(* Logix 5000 AddOnInstructionDefinition export HI1769_AOI_INT; software revision 32.00; part 2 of 2 *)
(* tags used below, declared in another part *)
   Inp_hi1769 : HI:1769_xWS_ChannelNOCMD_r3:I:0;
   Out_hi1769 : HI:1769_xWS_Channel:O:0;
   cal_hi_cmd : BOOL;   // trigger the cal high command
   cal_low_cmd : BOOL;   // trigger the cal low command
   cmd_status : INT;
   cal_hi_ctrl : DINT;
   cal_lo_ctrl : DINT;
   CalHI_cmd_reset_timer : TIMER;
   CalLo_cmd_reset_timer : TIMER;
   Status_Return : HardyCmdResult;
(* HI1769_AOI_INT, continued *)

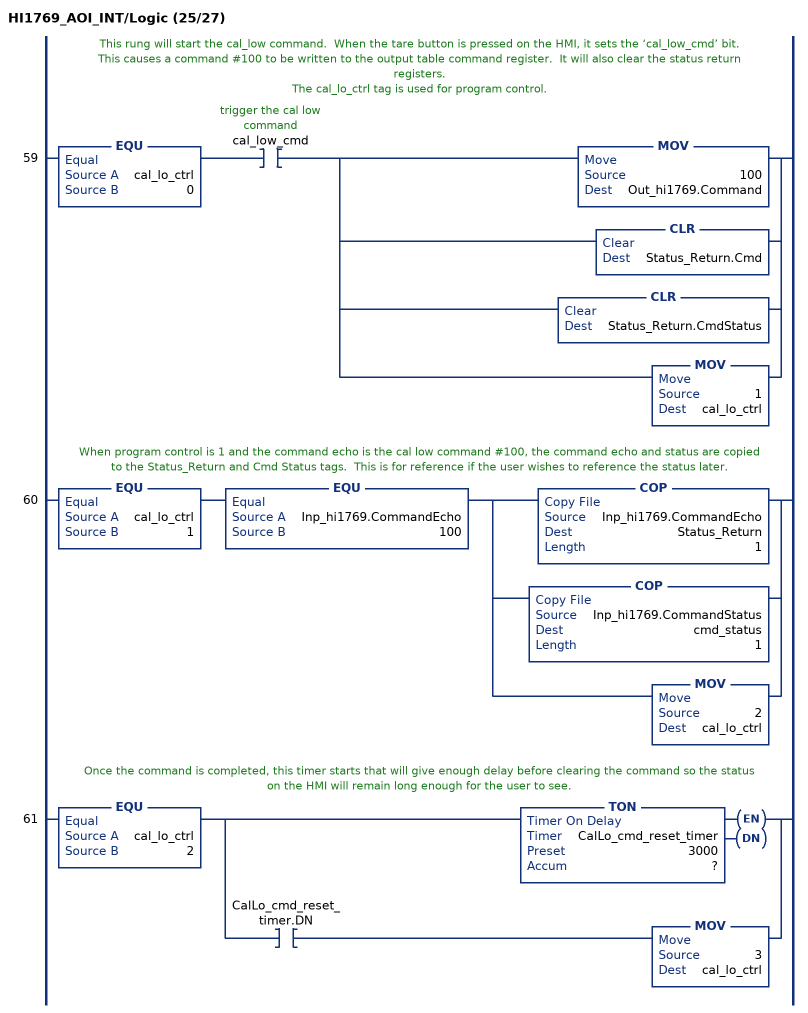
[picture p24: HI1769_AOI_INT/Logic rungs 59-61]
   // This rung will start the cal_low command.  When the tare button is pressed on the HMI, it sets the ‘cal_low_cmd’ bit.
   // This causes a command #100 to be written to the output table command register.  It will also clear the status return registers.
   // The cal_lo_ctrl tag is used for program control.
   59: EQU(cal_lo_ctrl,0)XIC(cal_low_cmd)[MOV(100,Out_hi1769.Command) ,CLR(Status_Return.Cmd) ,CLR(Status_Return.CmdStatus) ,MOV(1,cal_lo_ctrl) ];
   // When program control is 1 and the command echo is the cal low command #100, the command echo and status are copied to the Status_Return and Cmd Status tags.  This is for reference if the user wishes to reference the status later.
   60: EQU(cal_lo_ctrl,1)EQU(Inp_hi1769.CommandEcho,100)[COP(Inp_hi1769.CommandEcho,Status_Return,1) ,COP(Inp_hi1769.CommandStatus,cmd_status,1) ,MOV(2,cal_lo_ctrl) ];
   // Once the command is completed, this timer starts that will give enough delay before clearing the command so the status on the HMI will remain long enough for the user to see.
   61: EQU(cal_lo_ctrl,2)[TON(CalLo_cmd_reset_timer,?,?) ,XIC(CalLo_cmd_reset_timer.DN) MOV(3,cal_lo_ctrl) ];
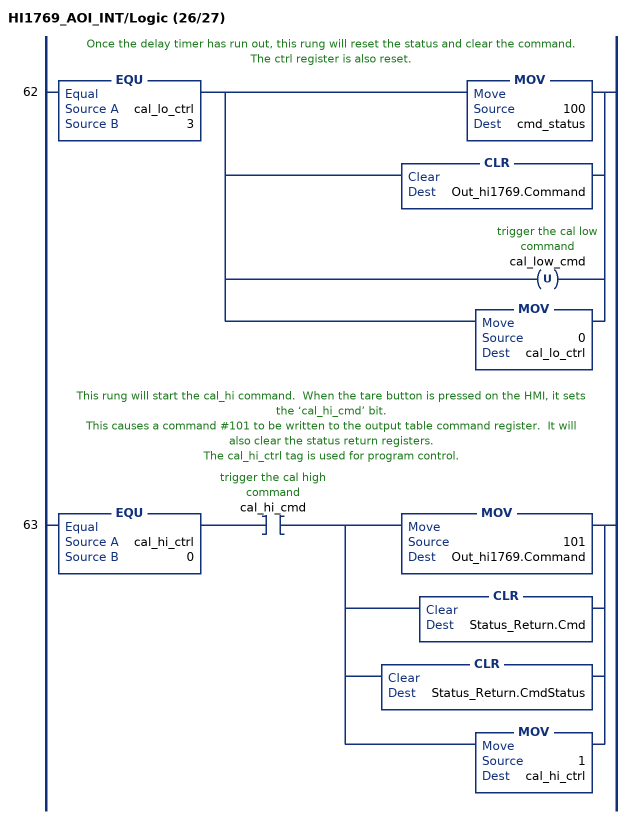
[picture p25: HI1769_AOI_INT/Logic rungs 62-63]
   // Once the delay timer has run out, this rung will reset the status and clear the command.
   // The ctrl register is also reset.
   62: EQU(cal_lo_ctrl,3)[MOV(100,cmd_status) ,CLR(Out_hi1769.Command) ,OTU(cal_low_cmd) ,MOV(0,cal_lo_ctrl) ];
   // This rung will start the cal_hi command.  When the tare button is pressed on the HMI, it sets the ‘cal_hi_cmd’ bit.
   // This causes a command #101 to be written to the output table command register.  It will also clear the status return registers.
   // The cal_hi_ctrl tag is used for program control.
   63: EQU(cal_hi_ctrl,0)XIC(cal_hi_cmd)[MOV(101,Out_hi1769.Command) ,CLR(Status_Return.Cmd) ,CLR(Status_Return.CmdStatus) ,MOV(1,cal_hi_ctrl) ];
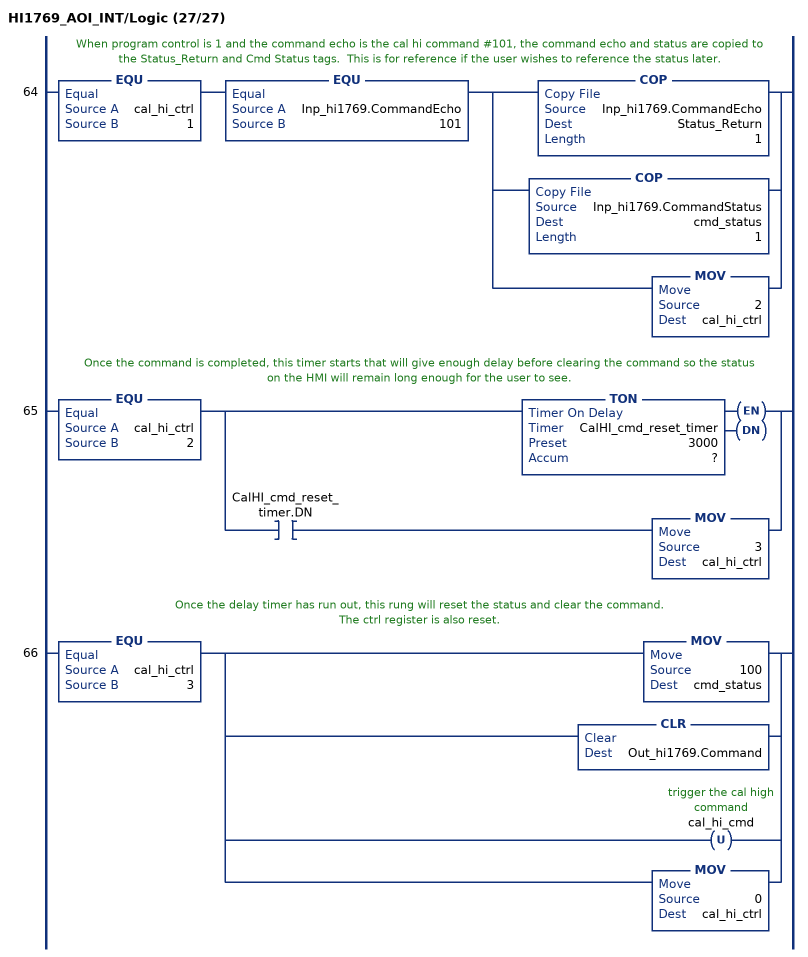
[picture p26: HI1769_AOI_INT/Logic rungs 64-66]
   // When program control is 1 and the command echo is the cal hi command #101, the command echo and status are copied to the Status_Return and Cmd Status tags.  This is for reference if the user wishes to reference the status later.
   64: EQU(cal_hi_ctrl,1)EQU(Inp_hi1769.CommandEcho,101)[COP(Inp_hi1769.CommandEcho,Status_Return,1) ,COP(Inp_hi1769.CommandStatus,cmd_status,1) ,MOV(2,cal_hi_ctrl) ];
   // Once the command is completed, this timer starts that will give enough delay before clearing the command so the status on the HMI will remain long enough for the user to see.
   65: EQU(cal_hi_ctrl,2)[TON(CalHI_cmd_reset_timer,?,?) ,XIC(CalHI_cmd_reset_timer.DN) MOV(3,cal_hi_ctrl) ];
   // Once the delay timer has run out, this rung will reset the status and clear the command.
   // The ctrl register is also reset.
   66: EQU(cal_hi_ctrl,3)[MOV(100,cmd_status) ,CLR(Out_hi1769.Command) ,OTU(cal_hi_cmd) ,MOV(0,cal_hi_ctrl) ];
END_ROUTINE
END_ADD_ON_INSTRUCTION
